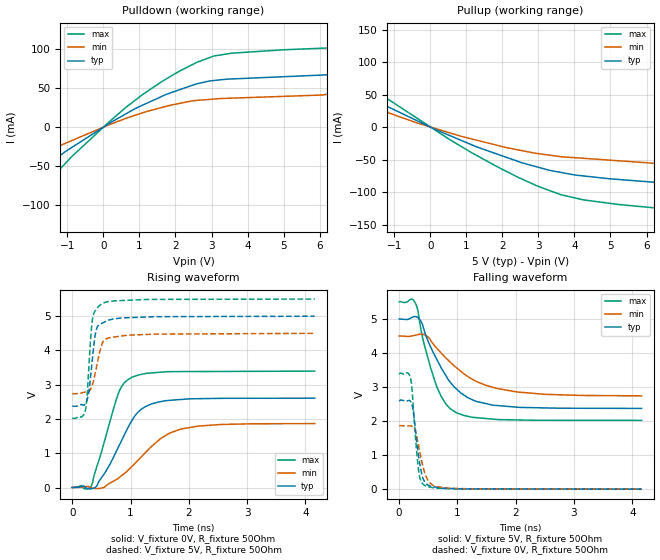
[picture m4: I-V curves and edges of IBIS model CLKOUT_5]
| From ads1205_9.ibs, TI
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|   CLKOUT OUTUPT 5V Model
[Model] CLKOUT_5
Model_type Output
|Signal CLKOUT
Polarity   Non-Inverting
Enable   Active-Low
Vmeas = 2.5
Vref = 2.5
Cref = 15pF
Rref = 50
|   typ   min   max
|   AVERAGE
C_comp   1.6450350e-12   1.5577160e-12   1.6845220e-12
|   OUTPUT HIGH
|C_comp   1.9276870e-12   1.8021110e-12   2.0979110e-12
|   OUTPUT LOW
|C_comp   1.2813210e-12   1.3133210e-12   1.2711330e-12
[Voltage Range]   5   4.5   5.5
[Temperature Range]   27   105   -40
[Pullup Reference]   5   4.5   5.5
[Pulldown Reference]   0   0   0
[Power Clamp Reference]   5   4.5   5.5
[GND Clamp Reference]   0   0   0
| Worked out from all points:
|   slope of the pulldown table from 0 to 0.75 V, typ, clamps not added: 36.7 ohm
|   slope of the pullup table from 0 to 0.75 V, typ, clamps not added: 41.7 ohm
|   falling waveform, V_fixture 5V, R_fixture 50Ohm: 20-80 % time 545ps typ, 787ps min, 363ps max; typ from 5 V to 2.37 V
|   rising waveform, V_fixture 0V, R_fixture 50Ohm: 20-80 % time 480ps typ, 710ps min, 351ps max; typ from 0 V to 2.61 V
|   rising waveform, V_fixture 5V, R_fixture 50Ohm: 20-80 % time 104ps typ, 140ps min, 82.6ps max; typ from 2.37 V to 5 V
|   falling waveform, V_fixture 0V, R_fixture 50Ohm: 20-80 % time 121ps typ, 154ps min, 94.9ps max; typ from 2.61 V to 0 V
[Pulldown]
|   Voltage   I(typ)   I(min)   I(max)
-5V       -314mA     -182.9mA   -547.6mA
-3.356V   -162.6mA   -92.61mA   -289.7mA
-3.007V   -130.4mA   -74.98mA   -234.9mA
-2.347V   -82.68mA   -53.44mA   -133.1mA
-1.365V   -42.01mA   -27.33mA   -61.6mA
144.6mV   4.186mA    2.732mA    6.192mA
2.625V    55.97mA    34.42mA    83.79mA
3.546V    61.82mA    37.17mA    94.83mA
6.642V    68.46mA    44.9mA     102.4mA
7.365V    79.68mA    69.3mA     108.1mA
7.925V    127.4mA    100.7mA    149.1mA
9.985V    321.7mA    217.9mA    478.3mA
[Pullup]
|   Voltage   I(typ)   I(min)   I(max)
-5V       322.4mA    190.5mA    557.9mA
-2.911V   125.3mA    72.1mA     223.6mA
-2.582V   94.32mA    56.79mA    171mA
-2.365V   75.68mA    49.99mA    136.2mA
-2.003V   57.63mA    40.67mA    83.27mA
-1.493V   39.76mA    28.58mA    54.57mA
2.967V    -61.23mA   -40.45mA   -90.44mA
4.242V    -74.97mA   -47.87mA   -111.7mA
6.617V    -86.63mA   -60.26mA   -126.1mA
7.755V    -116.5mA   -88.98mA   -155.8mA
8.278V    -157.7mA   -116.5mA   -204.7mA
9.985V    -314.7mA   -210.5mA   -471.5mA
[Ramp]
R_load = 50
|   typ   min   max
dV/dt_r   1.564/4.77866e-10   1.11951/6.99739e-10   2.03799/3.4828e-10
dV/dt_f   1.57666/5.41894e-10   1.05564/7.83949e-10   2.0878/3.62261e-10
[Falling Waveform]
V_fixture = 5V
V_fixture_min = 4.5V
V_fixture_max = 5.5V
R_fixture = 50Ohm
C_fixture = 0F
|   Time   V(typ)   V(min)   V(max)
0s        5V         4.5V       5.5V
274.6ps   5.072V     4.522V     5.479V
323.1ps   5.037V     4.54V      5.239V
396.9ps   4.853V     4.551V     4.499V
636.3ps   3.844V     4.156V     3.05V
802.8ps   3.332V     3.851V     2.5V
980.9ps   2.947V     3.569V     2.248V
1.321ns   2.579V     3.168V     2.101V
2.023ns   2.408V     2.855V     2.034V
4.161ns   2.372V     2.741V     2.02V
[Rising Waveform]
V_fixture = 0V
V_fixture_min = 0V
V_fixture_max = 0V
R_fixture = 50Ohm
C_fixture = 0F
|   Time   V(typ)   V(min)   V(max)
0s        1.008nV    4.516nV    905.8pV
324.6ps   -35.63mV   -10.33mV   32.44mV
414.3ps   28.53mV    -33.79mV   569.9mV
795.9ps   1.195V     280.1mV    2.77V
887.8ps   1.516V     400.3mV    3.046V
1.022ns   1.952V     610mV      3.214V
1.174ns   2.271V     875.4mV    3.299V
1.341ns   2.427V     1.17V      3.342V
1.885ns   2.572V     1.713V     3.383V
4.161ns   2.607V     1.866V     3.397V
[Rising Waveform]
V_fixture = 5V
V_fixture_min = 4.5V
V_fixture_max = 5.5V
R_fixture = 50Ohm
C_fixture = 0F
|   Time   V(typ)   V(min)   V(max)
0s        2.372V     2.737V     2.02V
221.2ps   2.432V     2.784V     2.22V
253.3ps   2.549V     2.775V     2.656V
283.3ps   2.788V     2.796V     3.475V
316.8ps   3.281V     2.88V      4.379V
347.3ps   3.791V     3.012V     4.917V
411ps     4.599V     3.48V      5.195V
516.7ps   4.8V       4.218V     5.375V
938.5ps   4.954V     4.444V     5.463V
4.161ns   5V         4.5V       5.5V
[Falling Waveform]
|Gnd
V_fixture = 0V
V_fixture_min = 0V
V_fixture_max = 0V
R_fixture = 50Ohm
C_fixture = 0F
|   Time   V(typ)   V(min)   V(max)
0s        2.607V     1.867V     3.397V
197.9ps   2.572V     1.858V     3.247V
242ps     2.3V       1.828V     2.428V
288.1ps   1.627V     1.647V     1.351V
338.9ps   917mV      1.226V     483.6mV
389.7ps   434.4mV    799mV      188.9mV
457ps     171.8mV    391.9mV    89.68mV
571.3ps   74.91mV    123.1mV    46.29mV
849.8ps   22.44mV    29.28mV    14.57mV
4.161ns   3.678uV    36.38uV    291.4nV
